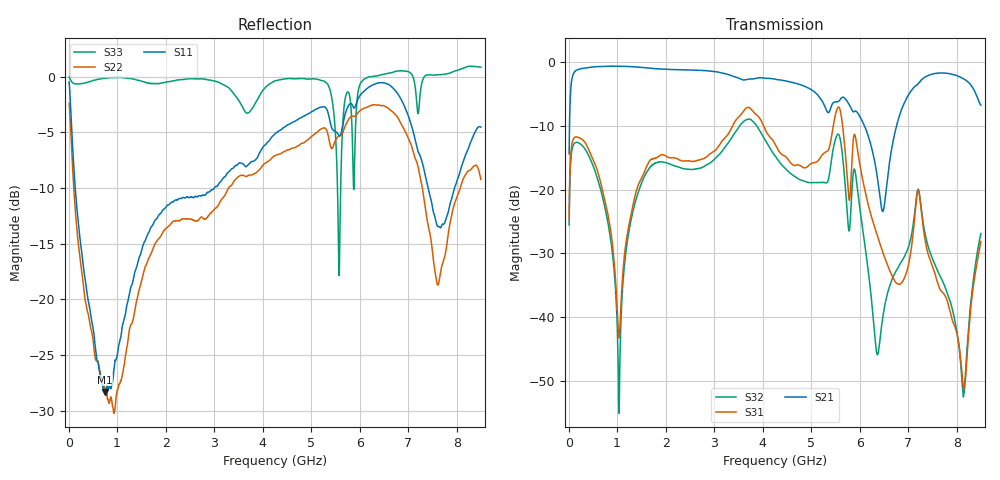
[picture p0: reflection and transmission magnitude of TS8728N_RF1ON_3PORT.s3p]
!Created with skrf (http://scikit-rf.org).
# GHz S RI R 50.0
!freq ReS11 ImS11 ReS12 ImS12 ReS13 ImS13
! ReS21 ImS21 ReS22 ImS22 ReS23 ImS23
! ReS31 ImS31 ReS32 ImS32 ReS33 ImS33
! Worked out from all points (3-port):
!   1601 points, 10 MHz to 8.5 GHz, reference 50 ohm
!   strongest paths, dB at 10 MHz, 2.132 GHz, 4.255 GHz, 6.378 GHz, 8.5 GHz:
!     S21: -14.4, -1.2, -2.7, -18.7, -6.7
!     S31: -24.6, -15.0, -12.8, -27.5, -28.1
!     S32: -25.5, -16.1, -14.7, -45.7, -26.9
!   lowest |S11| = -28.3 dB at 742.3 MHz (marker M1), VSWR 1.08, Z = 53.8 + j1.1 ohm
!   |S11| at or under -10 dB: 135.9 MHz to 3.001 GHz (2.865 GHz wide, 183 % of centre); 7.412 GHz to 7.954 GHz (541.5 MHz wide, 7.05 % of centre)
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0.01  -0.9243 0.2014  0.0688 0.1784  0.0147 0.057
      0.0688 0.1783  -0.7404 0.1669  0.0134 0.0512
      0.0148 0.057  0.0134 0.0513  -0.9922 0.06
0.7422625  0.0371 0.0102  0.906 -0.1958  0.0191 -0.0817
           0.9061 -0.1959  0.0393 0.0092  0.00324 -0.0743
           0.0191 -0.0817  0.00325 -0.0742  0.9089 0.3721
1.039413  0.0293 -0.0557  0.8697 -0.3269  0.00681 -0.000955
          0.8695 -0.3268  0.0176 -0.0379  -0.00166 0.000588
          0.00681 -0.000997  -0.00166 0.000607  0.9896 -0.0552
1.564731  -0.0504 -0.1742  0.7445 -0.514  0.1057 0.0895
          0.7446 -0.5139  -0.0776 -0.1126  0.1052 0.0719
          0.1055 0.0895  0.1055 0.0719  0.4718 -0.8187
3.114156  -0.2381 -0.2357  0.2537 -0.7897  0.2233 -0.0312
          0.2538 -0.7901  -0.2668 0.0571  0.168 -0.0898
          0.2229 -0.0312  0.1678 -0.0898  -0.5021 -0.792
4.255  -0.5145 -0.2049  -0.0858 -0.7302  -0.0516 -0.2225
       -0.0873 -0.7306  -0.3473 0.2732  -0.1046 -0.1514
       -0.0515 -0.2224  -0.1045 -0.152  0.0848 0.953
6.08035  -0.7826 0.3487  -0.2951 -0.1436  -0.0818 0.0755
         -0.295 -0.1433  0.3646 0.6186  -0.0201 0.039
         -0.0818 0.0754  -0.0202 0.0389  0.041 -0.9672
7.046087  -0.0229 0.6253  0.1676 -0.56  -0.015 0.0269
          0.1678 -0.561  0.4127 -0.2901  0.0016 -0.0402
          -0.015 0.027  0.00173 -0.04  1.026 -0.1536
8.139175  -0.3601 0.2097  -0.6161 -0.4122  0.00268 -0.000873
          -0.6164 -0.4115  0.0375 0.3468  0.00062 -0.00236
          0.00273 -0.000825  0.00057 -0.00231  -0.51 0.9626
8.5  -0.3429 0.4838  -0.3972 -0.2325  0.0226 0.0321
     -0.3972 -0.2322  0.3349 0.0848  0.0443 -0.0095
     0.0227 0.032  0.0444 -0.00947  -1.048 0.3332
